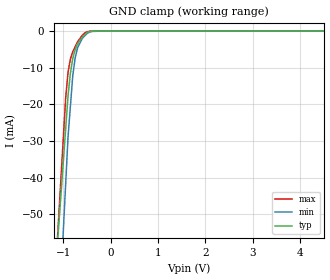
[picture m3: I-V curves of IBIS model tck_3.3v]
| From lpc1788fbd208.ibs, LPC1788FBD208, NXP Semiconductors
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[Model] tck_3.3v
Model_type Input
Vinl = 990.000mV
Vinh = 2.31000V
C_comp 983.000fF 934.000fF 1030.000fF
| variable typ   min   max
[Voltage Range] 3.30000V 3.00000V 3.60000V
[POWER Clamp Reference] 3.30000V 3.00000V 3.60000V
[GND Clamp Reference] 0.00000V 0.00000V 0.00000V
[Temperature Range]   25   85   -40
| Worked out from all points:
|   GND clamp passes 1 mA (typ) near -0.55 V on its own axis
[GND Clamp]
-3.3V     -450.8mA   -646.2mA   -536.1mA
-950mV    -26.65mA   -41.72mA   -18.28mA
-900mV    -17.63mA   -28.86mA   -11.23mA
-850mV    -11.48mA   -20.49mA   -7.604mA
-800mV    -7.48mA    -12.12mA   -5.625mA
-750mV    -5.083mA   -7.391mA   -4.288mA
-700mV    -3.587mA   -4.63mA    -2.952mA
-600mV    -1.67mA    -2.019mA   -1.153mA
-500mV    -451.2uA   -659.8uA   -172.8uA
-400mV    -39.9uA    -93.56uA   -28.06uA
-200mV    -2.5uA     -5.976uA   -2.038uA
6.6V      3.504uA    7.008uA    2.847uA
[POWER Clamp]
-3.3V     0A         0A         0A
6.6V      0A         0A         0A
